| TEXAS INSTRUMENTS INCORPORATED
| Standard Linear and Logic Group
| IBIS Model of SN74ALVCH16721
| 3.3V 20-Bit Flip-Flop with 3-state outputs
| This file contains package information for the following:
|  SSOP 56-pin (DL) package as [Component] ALVCH16721_DL
|  TSSOP 56-pin (DGG) package as [Component] ALVCH16721_DGG
|  TVSOP 56-pin (DGV) package as [Component] ALVCH16721_DGV
| This device can be powered at the following Vccs:
|  1.8 volt Vcc
|  2.5 volt Vcc
|  3.3 volt Vcc
|  2.7 volt Vcc
| This file provides unique models under the [Model Selector] for each Vcc.
| For operation at a specific Vcc, select the appropriate model after each
| [Model Selector] keyword.
[IBIS Ver]   3.2
[Comment char]  |_char
[File Name]   sn74alvch16721.ibs
[File Rev]   1.1 | b_die
[Date]   April 25, 2005
[Source]   Data created from TI-SPICE simulations at TI-SLL.
[Notes]   The following is an IBIS list for the ALVCH16721.
   Please contact sllibis@ti.com with questions and
   comments concerning SLL IBIS models.
   This IBIS model is created from a BA (back annotated netlist)
   - FILE REV HISTORY
   - 1.1 Release IBIS file on 04/26/05
   - Non-monotonic data in ground-clamp due to bus-hold
[Disclaimer] Property of Texas Instruments Incorporated.  Unauthorized
   reproduction and/or distribution is strictly prohibited.
   This product is protected under copyright law.
   Created  2005, (C) Copyright  2005, Texas Instruments
   Incorporated, All Rights Reserved
   UNLESS THERE IS A SIGNED, WRITTEN AGREEMENT TO THE
   CONTRARY, TEXAS INSTRUMENTS (TI) IS PROVIDING THE IBIS
   MODELS  AND WITHOUT ANY WARRANTY, EXPRESSED OR
   IMPLIED.  TI assumes no liability for:
   1) the accuracy of the IBIS models provided to your
   company;
   2) the proper functioning of these IBIS Models in your
   design or for any resulting applications; or
   3) infringement of patents, copyrights or intellectual
   property rights resulting from your use of these IBIS
   models.
   TI provides IBIS Models as a service to our customers.
   You and your company shall not distribute, sell or give
   these models to anyone else without prior written
   permission from TI.
   TI reserves the right to make changes to our products or
   to discontinue any semiconductor product or service
   without notice, and advises our customers to obtain the
   latest version of relevant information to verify, before
   placing orders, that the information being relied on is
   current.
   Please be aware that your receipt and use of the IBIS
   information provided shall serve as acceptance of these
   terms and conditions.  If you do not accept these terms,
   you should return or destroy the IBIS models and any
   other accompanying information immediately.
| Component ALVCH16721_DL 56-pin SSOP
[Component]   ALVCH16721_DL
[Manufacturer]   Texas Instruments, Inc.
[Package]
|   typ   min   max
R_pkg   5.500e-02   4.800e-02   6.700e-02
L_pkg   6.539e-09   4.803e-09   9.746e-09
C_pkg   8.570e-13   5.000e-13   1.351e-12
[Pin]   signal_name   model_name   R_pin   L_pin   C_pin
1   NOE   ALVCH16721_OE   6.400e-02   9.646e-09   1.202e-12
2   Q1   ALVCH16721_OUT   5.900e-02   8.723e-09   1.348e-12
3   Q2   ALVCH16721_OUT   5.900e-02   8.139e-09   1.223e-12
4   GND   GND   5.600e-02   7.554e-09   1.088e-12
5   Q3   ALVCH16721_OUT   5.400e-02   6.991e-09   9.660e-13
6   Q4   ALVCH16721_OUT   5.300e-02   6.659e-09   9.730e-13
7   VCC   POWER   5.500e-02   6.321e-09   9.050e-13
8   Q5   ALVCH16721_OUT   5.600e-02   5.942e-09   7.130e-13
9   Q6   ALVCH16721_OUT   5.700e-02   5.768e-09   6.780e-13
10   Q7   ALVCH16721_OUT   5.400e-02   5.459e-09   6.310e-13
11   GND   GND   5.100e-02   5.224e-09   6.380e-13
12   Q8   ALVCH16721_OUT   4.800e-02   5.088e-09   6.010e-13
13   Q9   ALVCH16721_OUT   5.000e-02   5.021e-09   5.180e-13
14   Q10   ALVCH16721_OUT   5.100e-02   4.803e-09   5.000e-13
15   Q11   ALVCH16721_OUT   5.100e-02   4.803e-09   5.000e-13
16   Q12   ALVCH16721_OUT   5.000e-02   5.021e-09   5.180e-13
17   Q13   ALVCH16721_OUT   4.800e-02   5.088e-09   6.010e-13
18   GND   GND   5.100e-02   5.224e-09   6.380e-13
19   Q14   ALVCH16721_OUT   5.400e-02   5.459e-09   6.310e-13
20   Q15   ALVCH16721_OUT   5.700e-02   5.768e-09   6.770e-13
21   Q16   ALVCH16721_OUT   5.500e-02   5.942e-09   7.150e-13
22   VCC   POWER   5.500e-02   6.321e-09   9.070e-13
23   Q17   ALVCH16721_OUT   5.300e-02   6.659e-09   9.720e-13
24   Q18   ALVCH16721_OUT   5.400e-02   6.991e-09   9.660e-13
25   GND   GND   5.600e-02   7.554e-09   1.087e-12
26   Q19   ALVCH16721_OUT   5.900e-02   8.139e-09   1.223e-12
27   Q20   ALVCH16721_OUT   5.900e-02   8.727e-09   1.351e-12
28   NC   NC   6.700e-02   9.746e-09   1.210e-12
29   NCLKEN   ALVCH16721_CE   6.300e-02   9.630e-09   1.203e-12
30   D20   ALVCH16721_IN   6.000e-02   8.751e-09   1.349e-12
31   D19   ALVCH16721_IN   6.000e-02   8.184e-09   1.224e-12
32   GND   GND   5.600e-02   7.543e-09   1.087e-12
33   D18   ALVCH16721_IN   5.400e-02   7.005e-09   9.690e-13
34   D17   ALVCH16721_IN   5.600e-02   6.714e-09   9.750e-13
35   VCC   POWER   5.800e-02   6.384e-09   9.090e-13
36   D16   ALVCH16721_IN   5.700e-02   5.976e-09   7.170e-13
37   D15   ALVCH16721_IN   5.700e-02   5.743e-09   6.770e-13
38   D14   ALVCH16721_IN   5.400e-02   5.468e-09   6.310e-13
39   GND   GND   5.500e-02   5.329e-09   6.440e-13
40   D13   ALVCH16721_IN   5.200e-02   5.189e-09   6.060e-13
41   D12   ALVCH16721_IN   5.200e-02   5.053e-09   5.190e-13
42   D11   ALVCH16721_IN   5.200e-02   4.825e-09   5.020e-13
43   D10   ALVCH16721_IN   5.400e-02   4.897e-09   5.060e-13
44   D9   ALVCH16721_IN   5.200e-02   5.093e-09   5.210e-13
45   D8   ALVCH16721_IN   5.100e-02   5.179e-09   6.080e-13
46   GND   GND   5.400e-02   5.314e-09   6.450e-13
47   D7   ALVCH16721_IN   5.500e-02   5.511e-09   6.320e-13
48   D6   ALVCH16721_IN   5.700e-02   5.770e-09   6.770e-13
49   D5   ALVCH16721_IN   5.600e-02   5.956e-09   7.160e-13
50   VCC   POWER   5.500e-02   6.320e-09   9.050e-13
51   D4   ALVCH16721_IN   5.200e-02   6.621e-09   9.680e-13
52   D3   ALVCH16721_IN   5.300e-02   6.974e-09   9.660e-13
53   GND   GND   5.700e-02   7.571e-09   1.089e-12
54   D2   ALVCH16721_IN   5.700e-02   8.097e-09   1.219e-12
55   D1   ALVCH16721_IN   5.900e-02   8.723e-09   1.349e-12
56   CLK   ALVCH16721_CLK   6.100e-02   9.560e-09   1.199e-12
| Component ALVCH16721_DGG 56-pin TSSOP
[Component]   ALVCH16721_DGG
[Manufacturer]   Texas Instruments, Inc.
[Package]
|   typ   min   max
R_pkg   4.500e-02   3.500e-02   6.200e-02
L_pkg   3.324e-09   2.403e-09   5.094e-09
C_pkg   5.640e-13   3.410e-13   9.140e-13
[Pin]   signal_name   model_name   R_pin   L_pin   C_pin
1   NOE   ALVCH16721_OE   6.200e-02   5.094e-09   8.560e-13
2   Q1   ALVCH16721_OUT   6.100e-02   4.621e-09   9.020e-13
3   Q2   ALVCH16721_OUT   6.000e-02   4.316e-09   8.020e-13
4   GND   GND   5.900e-02   3.968e-09   6.980e-13
5   Q3   ALVCH16721_OUT   5.700e-02   3.716e-09   6.490e-13
6   Q4   ALVCH16721_OUT   4.200e-02   3.517e-09   6.530e-13
7   VCC   POWER   4.100e-02   3.160e-09   5.700e-13
8   Q5   ALVCH16721_OUT   3.900e-02   2.981e-09   4.820e-13
9   Q6   ALVCH16721_OUT   3.900e-02   2.808e-09   4.470e-13
10   Q7   ALVCH16721_OUT   3.800e-02   2.715e-09   4.090e-13
11   GND   GND   4.100e-02   2.675e-09   3.910e-13
12   Q8   ALVCH16721_OUT   3.900e-02   2.536e-09   3.660e-13
13   Q9   ALVCH16721_OUT   3.900e-02   2.457e-09   3.480e-13
14   Q10   ALVCH16721_OUT   3.800e-02   2.411e-09   3.530e-13
15   Q11   ALVCH16721_OUT   3.900e-02   2.456e-09   3.550e-13
16   Q12   ALVCH16721_OUT   3.900e-02   2.471e-09   3.490e-13
17   Q13   ALVCH16721_OUT   4.000e-02   2.580e-09   3.700e-13
18   GND   GND   3.800e-02   2.651e-09   3.890e-13
19   Q14   ALVCH16721_OUT   3.800e-02   2.739e-09   4.110e-13
20   Q15   ALVCH16721_OUT   3.900e-02   2.838e-09   4.490e-13
21   Q16   ALVCH16721_OUT   3.800e-02   2.988e-09   4.840e-13
22   VCC   POWER   3.800e-02   3.104e-09   5.640e-13
23   Q17   ALVCH16721_OUT   4.000e-02   3.427e-09   6.380e-13
24   Q18   ALVCH16721_OUT   5.600e-02   3.654e-09   6.410e-13
25   GND   GND   5.700e-02   3.932e-09   7.000e-13
26   Q19   ALVCH16721_OUT   5.800e-02   4.257e-09   8.060e-13
27   Q20   ALVCH16721_OUT   5.700e-02   4.580e-09   9.140e-13
28   NC   NC   5.900e-02   5.038e-09   8.610e-13
29   NCLKEN   ALVCH16721_CE   6.000e-02   5.058e-09   8.580e-13
30   D20   ALVCH16721_IN   5.600e-02   4.543e-09   9.040e-13
31   D19   ALVCH16721_IN   5.700e-02   4.241e-09   8.020e-13
32   GND   GND   5.900e-02   3.933e-09   6.990e-13
33   D18   ALVCH16721_IN   5.600e-02   3.616e-09   6.370e-13
34   D17   ALVCH16721_IN   3.700e-02   3.368e-09   6.400e-13
35   VCC   POWER   3.600e-02   3.024e-09   5.630e-13
36   D16   ALVCH16721_IN   3.500e-02   2.876e-09   4.740e-13
37   D15   ALVCH16721_IN   3.500e-02   2.745e-09   4.440e-13
38   D14   ALVCH16721_IN   3.700e-02   2.683e-09   4.050e-13
39   GND   GND   3.800e-02   2.603e-09   3.820e-13
40   D13   ALVCH16721_IN   3.800e-02   2.510e-09   3.620e-13
41   D12   ALVCH16721_IN   3.600e-02   2.412e-09   3.410e-13
42   D11   ALVCH16721_IN   3.800e-02   2.416e-09   3.490e-13
43   D10   ALVCH16721_IN   3.800e-02   2.403e-09   3.490e-13
44   D9   ALVCH16721_IN   3.700e-02   2.429e-09   3.410e-13
45   D8   ALVCH16721_IN   3.600e-02   2.483e-09   3.580e-13
46   GND   GND   3.700e-02   2.614e-09   3.810e-13
47   D7   ALVCH16721_IN   3.500e-02   2.669e-09   4.020e-13
48   D6   ALVCH16721_IN   3.600e-02   2.763e-09   4.420e-13
49   D5   ALVCH16721_IN   3.600e-02   2.942e-09   4.780e-13
50   VCC   POWER   3.500e-02   3.053e-09   5.640e-13
51   D4   ALVCH16721_IN   3.600e-02   3.408e-09   6.410e-13
52   D3   ALVCH16721_IN   5.800e-02   3.698e-09   6.410e-13
53   GND   GND   5.900e-02   3.974e-09   6.970e-13
54   D2   ALVCH16721_IN   6.100e-02   4.327e-09   8.020e-13
55   D1   ALVCH16721_IN   6.100e-02   4.624e-09   9.050e-13
56   CLK   ALVCH16721_CLK   6.000e-02   5.063e-09   8.580e-13
| Component ALVCH16721_DGV 56-pin TVSOP
[Component]   ALVCH16721_DGV
[Manufacturer]   Texas Instruments, Inc.
[Package]
|   typ   min   max
R_pkg   6.300e-02   5.000e-02   8.400e-02
L_pkg   2.945e-09   2.394e-09   3.939e-09
C_pkg   3.910e-13   2.710e-13   5.880e-13
[Pin]   signal_name   model_name   R_pin   L_pin   C_pin
1   NOE   ALVCH16721_OE   6.800e-02   3.933e-09   5.880e-13
2   Q1   ALVCH16721_OUT   6.800e-02   3.568e-09   5.870e-13
3   Q2   ALVCH16721_OUT   7.600e-02   3.464e-09   5.150e-13
4   GND   GND   8.400e-02   3.444e-09   4.590e-13
5   Q3   ALVCH16721_OUT   8.100e-02   3.277e-09   4.270e-13
6   Q4   ALVCH16721_OUT   7.400e-02   3.136e-09   3.870e-13
7   VCC   POWER   6.900e-02   2.970e-09   4.010e-13
8   Q5   ALVCH16721_OUT   5.000e-02   2.785e-09   3.790e-13
9   Q6   ALVCH16721_OUT   5.100e-02   2.685e-09   3.200e-13
10   Q7   ALVCH16721_OUT   5.300e-02   2.611e-09   3.160e-13
11   GND   GND   5.300e-02   2.495e-09   2.970e-13
12   Q8   ALVCH16721_OUT   5.300e-02   2.435e-09   2.920e-13
13   Q9   ALVCH16721_OUT   5.500e-02   2.412e-09   2.850e-13
14   Q10   ALVCH16721_OUT   5.600e-02   2.401e-09   2.730e-13
15   Q11   ALVCH16721_OUT   5.500e-02   2.401e-09   2.730e-13
16   Q12   ALVCH16721_OUT   5.500e-02   2.399e-09   2.840e-13
17   Q13   ALVCH16721_OUT   5.400e-02   2.406e-09   2.890e-13
18   GND   GND   5.300e-02   2.450e-09   2.930e-13
19   Q14   ALVCH16721_OUT   5.100e-02   2.544e-09   3.110e-13
20   Q15   ALVCH16721_OUT   5.100e-02   2.626e-09   3.150e-13
21   Q16   ALVCH16721_OUT   5.000e-02   2.727e-09   3.690e-13
22   VCC   POWER   6.500e-02   2.903e-09   3.930e-13
23   Q17   ALVCH16721_OUT   7.500e-02   3.091e-09   3.860e-13
24   Q18   ALVCH16721_OUT   8.200e-02   3.272e-09   4.280e-13
25   GND   GND   8.200e-02   3.393e-09   4.570e-13
26   Q19   ALVCH16721_OUT   7.300e-02   3.380e-09   5.080e-13
27   Q20   ALVCH16721_OUT   7.100e-02   3.577e-09   5.800e-13
28   NC   NC   6.800e-02   3.937e-09   5.740e-13
29   NCLKEN   ALVCH16721_CE   6.900e-02   3.923e-09   5.690e-13
30   D20   ALVCH16721_IN   6.400e-02   3.536e-09   5.740e-13
31   D19   ALVCH16721_IN   7.600e-02   3.428e-09   5.170e-13
32   GND   GND   8.100e-02   3.395e-09   4.680e-13
33   D18   ALVCH16721_IN   8.000e-02   3.255e-09   4.310e-13
34   D17   ALVCH16721_IN   7.100e-02   3.064e-09   3.860e-13
35   VCC   POWER   6.100e-02   2.878e-09   3.890e-13
36   D16   ALVCH16721_IN   5.000e-02   2.710e-09   3.630e-13
37   D15   ALVCH16721_IN   5.000e-02   2.606e-09   3.110e-13
38   D14   ALVCH16721_IN   5.200e-02   2.534e-09   3.060e-13
39   GND   GND   5.200e-02   2.439e-09   2.890e-13
40   D13   ALVCH16721_IN   5.300e-02   2.399e-09   2.860e-13
41   D12   ALVCH16721_IN   5.500e-02   2.394e-09   2.820e-13
42   D11   ALVCH16721_IN   5.500e-02   2.398e-09   2.710e-13
43   D10   ALVCH16721_IN   5.600e-02   2.396e-09   2.710e-13
44   D9   ALVCH16721_IN   5.400e-02   2.402e-09   2.830e-13
45   D8   ALVCH16721_IN   5.400e-02   2.423e-09   2.880e-13
46   GND   GND   5.300e-02   2.474e-09   2.920e-13
47   D7   ALVCH16721_IN   5.100e-02   2.569e-09   3.090e-13
48   D6   ALVCH16721_IN   5.100e-02   2.638e-09   3.130e-13
49   D5   ALVCH16721_IN   5.100e-02   2.742e-09   3.660e-13
50   VCC   POWER   6.400e-02   2.917e-09   3.900e-13
51   D4   ALVCH16721_IN   7.400e-02   3.083e-09   3.830e-13
52   D3   ALVCH16721_IN   8.100e-02   3.249e-09   4.300e-13
53   GND   GND   8.300e-02   3.400e-09   4.550e-13
54   D2   ALVCH16721_IN   7.500e-02   3.427e-09   5.050e-13
55   D1   ALVCH16721_IN   7.100e-02   3.585e-09   5.780e-13
56   CLK   ALVCH16721_CLK   6.900e-02   3.939e-09   5.810e-13
| Model ALVCH16721_CE
[Model Selector]   ALVCH16721_CE
ALVCH16721_CE_18   1.8 volt Vcc
ALVCH16721_CE_25   2.5 volt Vcc
ALVCH16721_CE_33   3.3 volt Vcc
ALVCH16721_CE_27   2.7 volt Vcc
| Model ALVCH16721_OE
[Model Selector]   ALVCH16721_OE
ALVCH16721_OE_18   1.8 volt Vcc
ALVCH16721_OE_25   2.5 volt Vcc
ALVCH16721_OE_33   3.3 volt Vcc
ALVCH16721_OE_27   2.7 volt Vcc
| Model ALVCH16721_CLK
[Model Selector]   ALVCH16721_CLK
ALVCH16721_CLK_18   1.8 volt Vcc
ALVCH16721_CLK_25   2.5 volt Vcc
ALVCH16721_CLK_33   3.3 volt Vcc
ALVCH16721_CLK_27   2.7 volt Vcc
| Model ALVCH16721_IN
[Model Selector]   ALVCH16721_IN
ALVCH16721_IN_18   1.8 volt Vcc
ALVCH16721_IN_25   2.5 volt Vcc
ALVCH16721_IN_33   3.3 volt Vcc
ALVCH16721_IN_27   2.7 volt Vcc
| Model ALVCH16721_OUT
[Model Selector]   ALVCH16721_OUT
ALVCH16721_OUT_18   1.8 volt Vcc
ALVCH16721_OUT_25   2.5 volt Vcc
ALVCH16721_OUT_33   3.3 volt Vcc
ALVCH16721_OUT_27   2.7 volt Vcc
| Models and submodels in the file (20): ALVCH16721_CE_18 (Input), ALVCH16721_CE_25 (Input), ALVCH16721_CE_33 (Input), ALVCH16721_CE_27 (Input), ALVCH16721_OE_18 (Input), ALVCH16721_OE_25 (Input), ALVCH16721_OE_33 (Input), ALVCH16721_OE_27 (Input), ALVCH16721_CLK_18 (Input), ALVCH16721_CLK_25 (Input), ALVCH16721_CLK_33 (Input), ALVCH16721_CLK_27 (Input), ALVCH16721_IN_18 (Input), ALVCH16721_IN_25 (Input), ALVCH16721_IN_33 (Input), ALVCH16721_IN_27 (Input), ALVCH16721_OUT_18 (3-state), ALVCH16721_OUT_25 (3-state), ALVCH16721_OUT_33 (3-state), ALVCH16721_OUT_27 (3-state)
